(* Logix 5000 AddOnInstructionDefinition export Banner_QS18COD_Param_v4; software revision 33.00; part 2 of 2 *)
(* tags used below, declared in another part *)
   QS18COD : Banner_QS18COD_v4;
   Port_Data : Banner_IOL_Port_v4;
   Port : DINT;
   Local_Control : DINT;
   Command_Being_Processed : BOOL;
   Update_Archive : BOOL;
   Index_Write_Inprocess : INT;
   Inprocess_Index : DINT;
(* Banner_QS18COD_Param_v4, continued *)

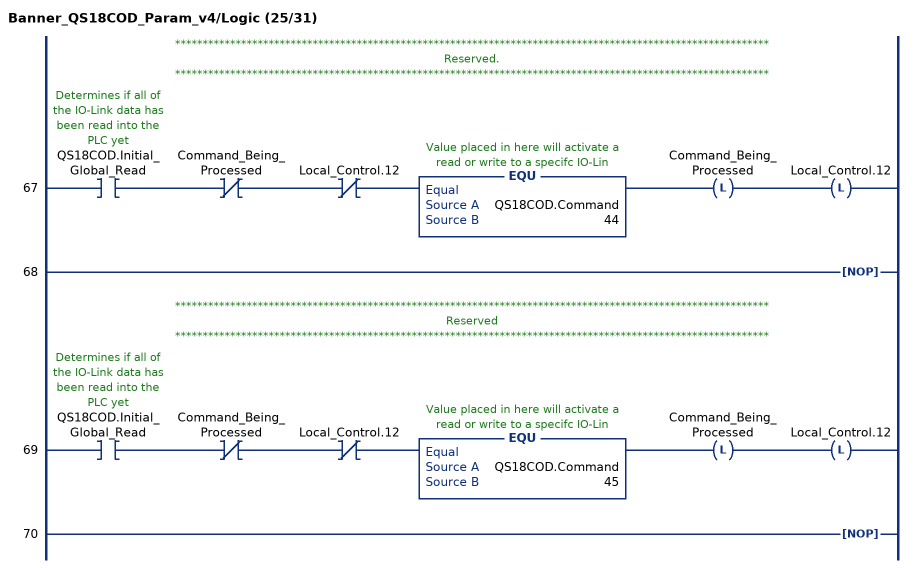
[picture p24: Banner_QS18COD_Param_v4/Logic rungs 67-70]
   // ************************************************************************************************************
   // Reserved.
   // ************************************************************************************************************
   67: XIC(QS18COD.Initial_Global_Read)XIO(Command_Being_Processed)XIO(Local_Control.12)EQU(QS18COD.Command,44)OTL(Command_Being_Processed)OTL(Local_Control.12);
   68: NOP();
   // ************************************************************************************************************
   // Reserved
   // ************************************************************************************************************
   69: XIC(QS18COD.Initial_Global_Read)XIO(Command_Being_Processed)XIO(Local_Control.12)EQU(QS18COD.Command,45)OTL(Command_Being_Processed)OTL(Local_Control.12);
   70: NOP();
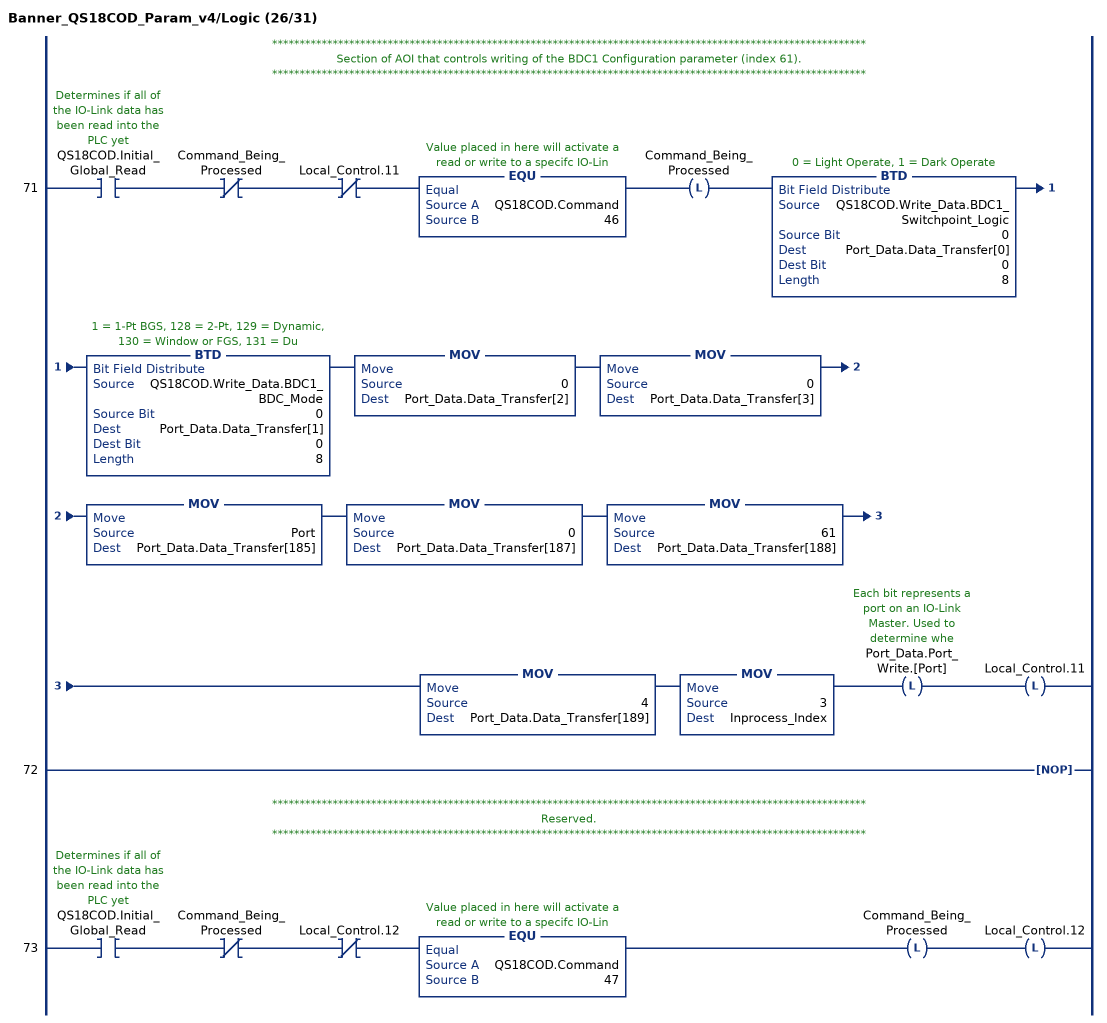
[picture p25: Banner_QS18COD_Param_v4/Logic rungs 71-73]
   // ************************************************************************************************************
   // Section of AOI that controls writing of the BDC1 Configuration parameter (index 61).
   // ************************************************************************************************************
   71: XIC(QS18COD.Initial_Global_Read)XIO(Command_Being_Processed)XIO(Local_Control.11)EQU(QS18COD.Command,46)OTL(Command_Being_Processed)BTD(QS18COD.Write_Data.BDC1_Switchpoint_Logic,0,Port_Data.Data_Transfer[0],0,8)BTD(QS18COD.Write_Data.BDC1_BDC_Mode,0,Port_Data.Data_Transfer[1],0,8)MOV(0,Port_Data.Data_Transfer[2])MOV(0,Port_Data.Data_Transfer[3])MOV(Port,Port_Data.Data_Transfer[185])MOV(0,Port_Data.Data_Transfer[187])MOV(61,Port_Data.Data_Transfer[188])MOV(4,Port_Data.Data_Transfer[189])MOV(3,Inprocess_Index)OTL(Port_Data.Port_Write.[Port])OTL(Local_Control.11);
   72: NOP();
   // ************************************************************************************************************
   // Reserved.
   // ************************************************************************************************************
   73: XIC(QS18COD.Initial_Global_Read)XIO(Command_Being_Processed)XIO(Local_Control.12)EQU(QS18COD.Command,47)OTL(Command_Being_Processed)OTL(Local_Control.12);
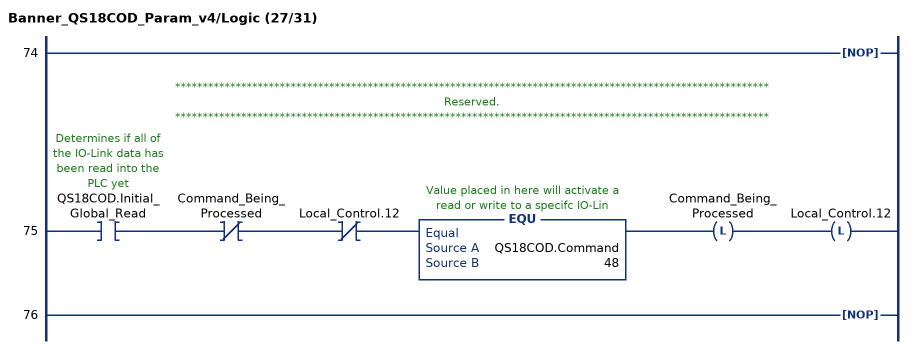
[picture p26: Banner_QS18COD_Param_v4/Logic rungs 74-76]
   74: NOP();
   // ************************************************************************************************************
   // Reserved.
   // ************************************************************************************************************
   75: XIC(QS18COD.Initial_Global_Read)XIO(Command_Being_Processed)XIO(Local_Control.12)EQU(QS18COD.Command,48)OTL(Command_Being_Processed)OTL(Local_Control.12);
   76: NOP();
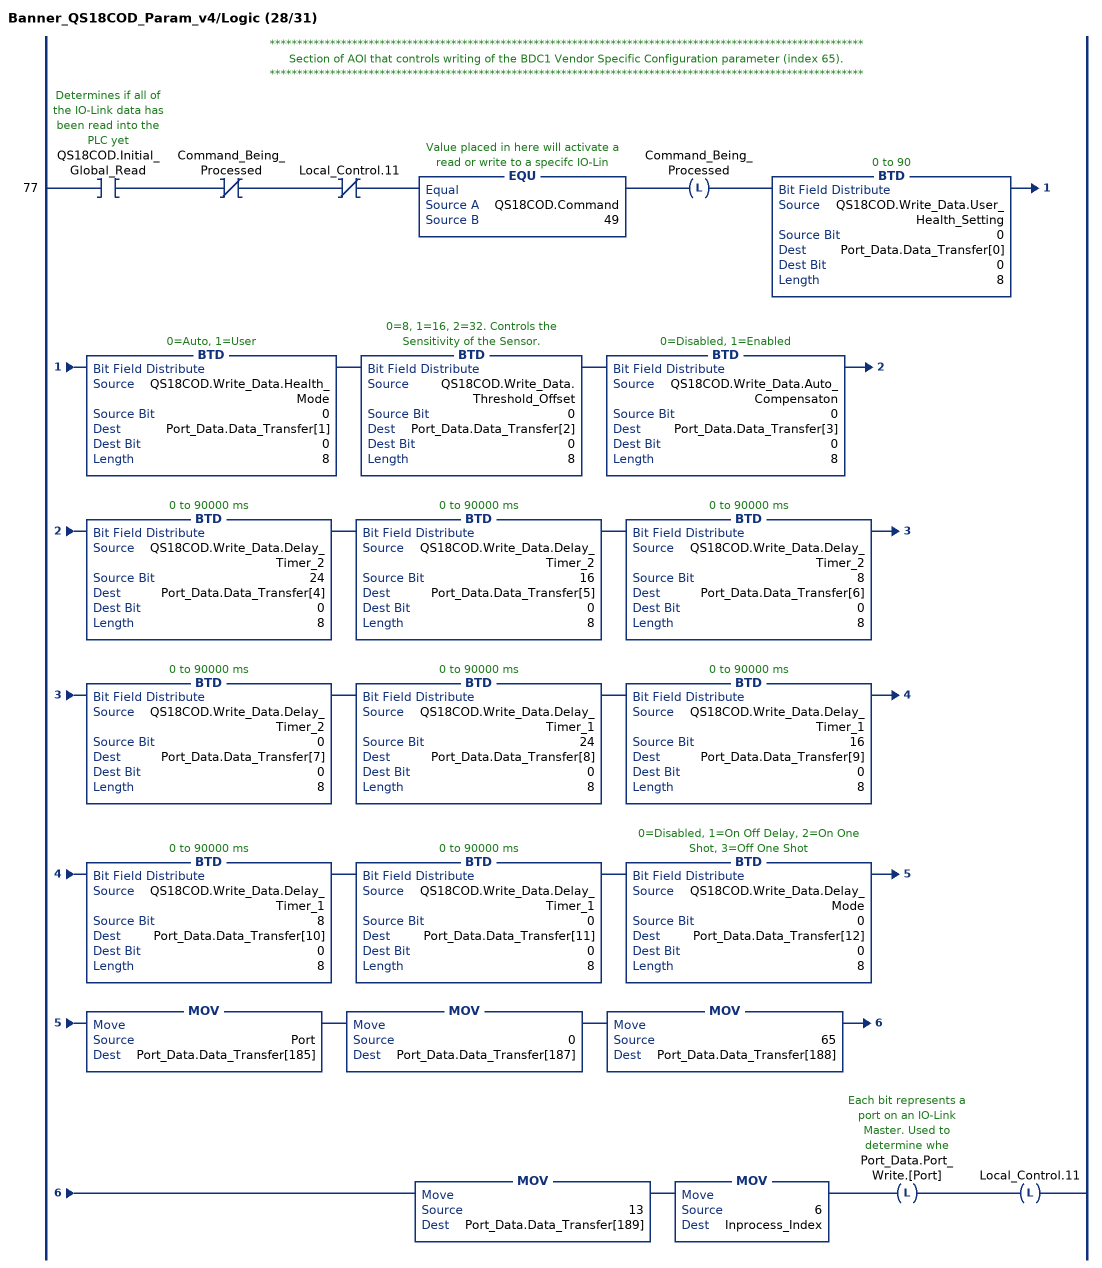
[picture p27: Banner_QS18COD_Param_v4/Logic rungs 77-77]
   // ************************************************************************************************************
   // Section of AOI that controls writing of the BDC1 Vendor Specific Configuration parameter (index 65).
   // ************************************************************************************************************
   77: XIC(QS18COD.Initial_Global_Read)XIO(Command_Being_Processed)XIO(Local_Control.11)EQU(QS18COD.Command,49)OTL(Command_Being_Processed)BTD(QS18COD.Write_Data.User_Health_Setting,0,Port_Data.Data_Transfer[0],0,8)BTD(QS18COD.Write_Data.Health_Mode,0,Port_Data.Data_Transfer[1],0,8)BTD(QS18COD.Write_Data.Threshold_Offset,0,Port_Data.Data_Transfer[2],0,8)BTD(QS18COD.Write_Data.Auto_Compensaton,0,Port_Data.Data_Transfer[3],0,8)BTD(QS18COD.Write_Data.Delay_Timer_2,24,Port_Data.Data_Transfer[4],0,8)BTD(QS18COD.Write_Data.Delay_Timer_2,16,Port_Data.Data_Transfer[5],0,8)BTD(QS18COD.Write_Data.Delay_Timer_2,8,Port_Data.Data_Transfer[6],0,8)BTD(QS18COD.Write_Data.Delay_Timer_2,0,Port_Data.Data_Transfer[7],0,8)BTD(QS18COD.Write_Data.Delay_Timer_1,24,Port_Data.Data_Transfer[8],0,8)BTD(QS18COD.Write_Data.Delay_Timer_1,16,Port_Data.Data_Transfer[9],0,8)BTD(QS18COD.Write_Data.Delay_Timer_1,8,Port_Data.Data_Transfer[10],0,8)BTD(QS18COD.Write_Data.Delay_Timer_1,0,Port_Data.Data_Transfer[11],0,8)BTD(QS18COD.Write_Data.Delay_Mode,0,Port_Data.Data_Transfer[12],0,8)MOV(Port,Port_Data.Data_Transfer[185])MOV(0,Port_Data.Data_Transfer[187])MOV(65,Port_Data.Data_Transfer[188])MOV(13,Port_Data.Data_Transfer[189])MOV(6,Inprocess_Index)OTL(Port_Data.Port_Write.[Port])OTL(Local_Control.11);
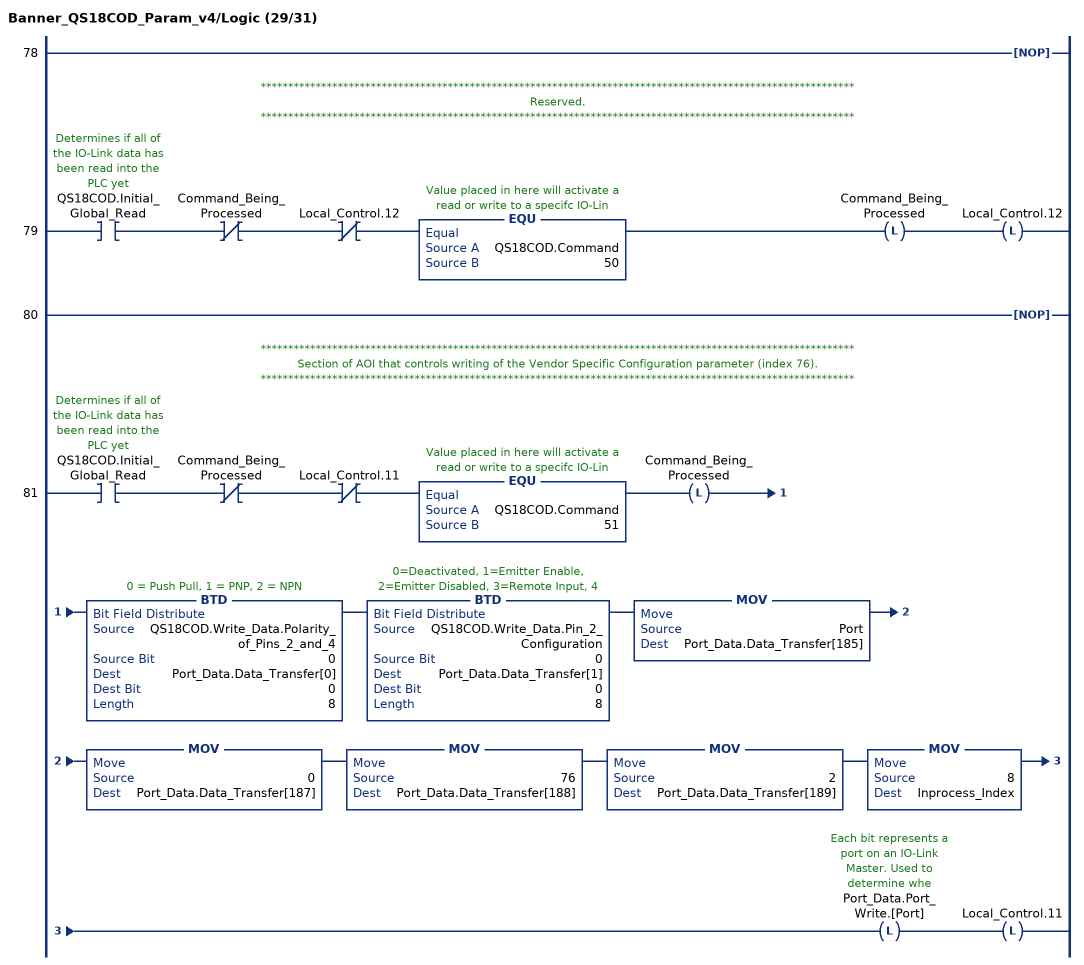
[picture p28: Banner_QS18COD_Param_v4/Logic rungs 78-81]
   78: NOP();
   // ************************************************************************************************************
   // Reserved.
   // ************************************************************************************************************
   79: XIC(QS18COD.Initial_Global_Read)XIO(Command_Being_Processed)XIO(Local_Control.12)EQU(QS18COD.Command,50)OTL(Command_Being_Processed)OTL(Local_Control.12);
   80: NOP();
   // ************************************************************************************************************
   // Section of AOI that controls writing of the Vendor Specific Configuration parameter (index 76).
   // ************************************************************************************************************
   81: XIC(QS18COD.Initial_Global_Read)XIO(Command_Being_Processed)XIO(Local_Control.11)EQU(QS18COD.Command,51)OTL(Command_Being_Processed)BTD(QS18COD.Write_Data.Polarity_of_Pins_2_and_4,0,Port_Data.Data_Transfer[0],0,8)BTD(QS18COD.Write_Data.Pin_2_Configuration,0,Port_Data.Data_Transfer[1],0,8)MOV(Port,Port_Data.Data_Transfer[185])MOV(0,Port_Data.Data_Transfer[187])MOV(76,Port_Data.Data_Transfer[188])MOV(2,Port_Data.Data_Transfer[189])MOV(8,Inprocess_Index)OTL(Port_Data.Port_Write.[Port])OTL(Local_Control.11);
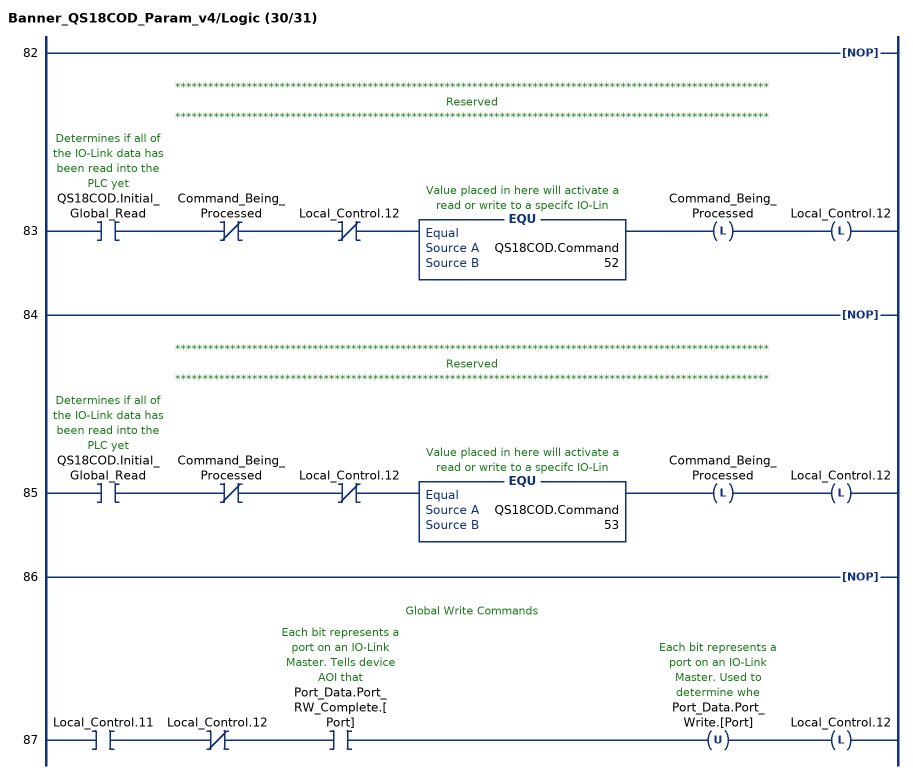
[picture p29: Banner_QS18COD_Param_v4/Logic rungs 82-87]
   82: NOP();
   // ************************************************************************************************************
   // Reserved
   // ************************************************************************************************************
   83: XIC(QS18COD.Initial_Global_Read)XIO(Command_Being_Processed)XIO(Local_Control.12)EQU(QS18COD.Command,52)OTL(Command_Being_Processed)OTL(Local_Control.12);
   84: NOP();
   // ************************************************************************************************************
   // Reserved
   // ************************************************************************************************************
   85: XIC(QS18COD.Initial_Global_Read)XIO(Command_Being_Processed)XIO(Local_Control.12)EQU(QS18COD.Command,53)OTL(Command_Being_Processed)OTL(Local_Control.12);
   86: NOP();
   // Global Write Commands
   87: XIC(Local_Control.11)XIO(Local_Control.12)XIC(Port_Data.Port_RW_Complete.[Port])OTU(Port_Data.Port_Write.[Port])OTL(Local_Control.12);
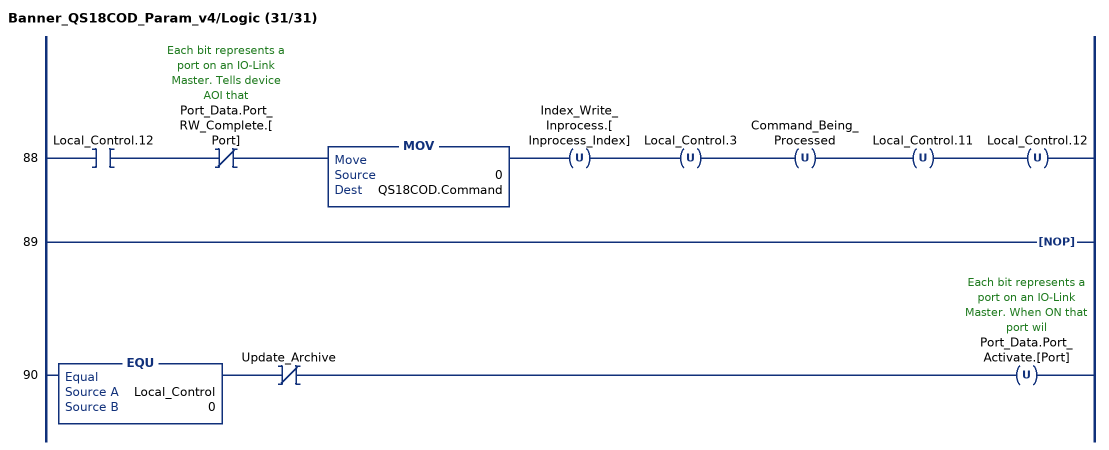
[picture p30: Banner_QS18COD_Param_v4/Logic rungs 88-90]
   88: XIC(Local_Control.12)XIO(Port_Data.Port_RW_Complete.[Port])MOV(0,QS18COD.Command)OTU(Index_Write_Inprocess.[Inprocess_Index])OTU(Local_Control.3)OTU(Command_Being_Processed)OTU(Local_Control.11)OTU(Local_Control.12);
   89: NOP();
   90: EQU(Local_Control,0)XIO(Update_Archive)OTU(Port_Data.Port_Activate.[Port]);
END_ROUTINE
END_ADD_ON_INSTRUCTION
